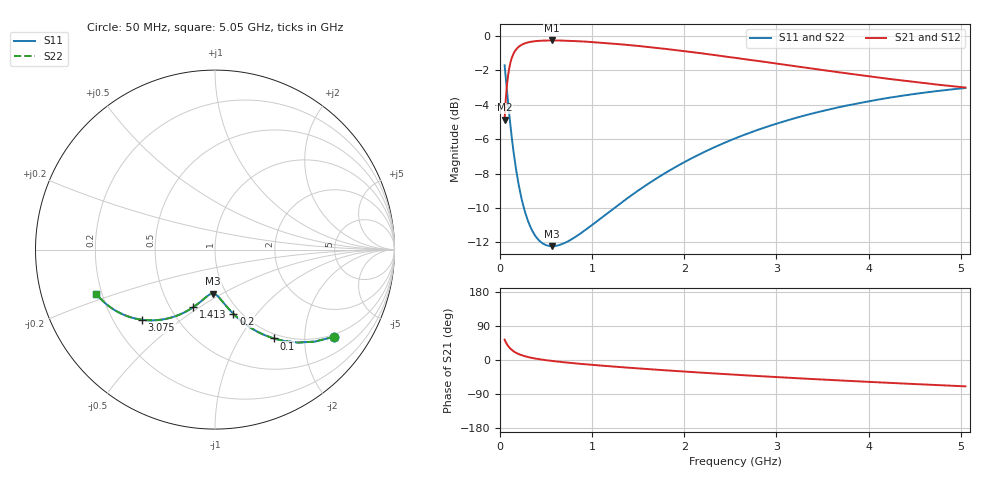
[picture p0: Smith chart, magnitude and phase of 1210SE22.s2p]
! AVX Thin Film Operation		Date: August 2001
! Description: Accu-P® Series, Thin Film, SMD, RF Capacitor
! Part Number: 12101J200FBT
! 50 MHz  -  5.05 GHz
! Serial Measurements
# mhz S db R 50
!	S11		S21		S12		S22
!	dB	Phase	dB	Phase	dB	Phase	dB	Phase
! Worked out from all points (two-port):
!   401 points, 50 MHz to 5.05 GHz, reference 50 ohm
!   highest |S21| = -0.27 dB at 562.5 MHz (marker M1); lowest = -4.9 dB at 50 MHz (marker M2)
!   |S21| within 3 dB of the highest: 69.04 MHz to end of sweep
!   lowest |S11| = -12.2 dB at 562.5 MHz (marker M3), VSWR 1.65, Z = 43.5 - j22.7 ohm
!   |S11| at or under -10 dB: 259.3 MHz to 1.24 GHz (980.7 MHz wide, 131 % of centre)
!   |S22| runs from -12.2 to -1.7 dB; largest |S21 - S12| = 0
!   S11 on the Smith chart (normalised r, x): 50 MHz: 0.93, -2.77; 100 MHz: 0.93, -1.42; 200 MHz: 0.92, -0.77; 1.413 GHz: 0.65, -0.47; 3.075 GHz: 0.32, -0.37; 5.05 GHz: 0.18, -0.18
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50  -1.71 -36.3  -4.87 53.7  -4.87 53.7  -1.71 -36.3
75  -3.15 -48.1  -2.88 41.9  -2.88 41.9  -3.15 -48.1
87.5  -3.86 -52.7  -2.31 37.3  -2.31 37.3  -3.86 -52.7
100  -4.54 -56.6  -1.89 33.4  -1.89 33.4  -4.54 -56.6
112.5  -5.18 -59.9  -1.57 30.1  -1.57 30.1  -5.18 -59.9
137.5  -6.34 -65.3  -1.15 24.7  -1.15 24.7  -6.34 -65.3
162.5  -7.34 -69.4  -0.89 20.6  -0.89 20.6  -7.34 -69.4
200  -8.57 -74.0  -0.65 15.9  -0.65 15.9  -8.57 -74.0
275  -10.30 -80.3  -0.43 9.6  -0.43 9.6  -10.30 -80.3
350  -11.32 -84.6  -0.33 5.4  -0.33 5.4  -11.32 -84.6
450  -12.01 -88.7  -0.28 1.2  -0.28 1.2  -12.01 -88.7
562.5  -12.22 -92.4  -0.27 -2.4  -0.27 -2.4  -12.22 -92.4
700  -12.04 -96.1  -0.28 -6.1  -0.28 -6.1  -12.04 -96.1
887.5  -11.43 -100.4  -0.33 -10.5  -0.33 -10.5  -11.43 -100.4
1412.5  -9.32 -110.6  -0.54 -20.6  -0.54 -20.6  -9.32 -110.6
1725  -8.20 -116.0  -0.72 -26.0  -0.72 -26.0  -8.20 -116.0
2125  -6.99 -122.4  -0.97 -32.5  -0.97 -32.5  -6.99 -122.4
2550  -5.96 -128.8  -1.27 -38.8  -1.27 -38.8  -5.96 -128.8
3075  -4.98 -136.1  -1.67 -46.1  -1.67 -46.1  -4.98 -136.1
3387.5  -4.51 -140.2  -1.90 -50.2  -1.90 -50.2  -4.52 -140.2
4225  -3.60 -150.3  -2.51 -60.3  -2.51 -60.3  -3.60 -150.3
5050  -3.03 -159.5  -3.00 -69.5  -3.00 -69.5  -3.03 -159.5
